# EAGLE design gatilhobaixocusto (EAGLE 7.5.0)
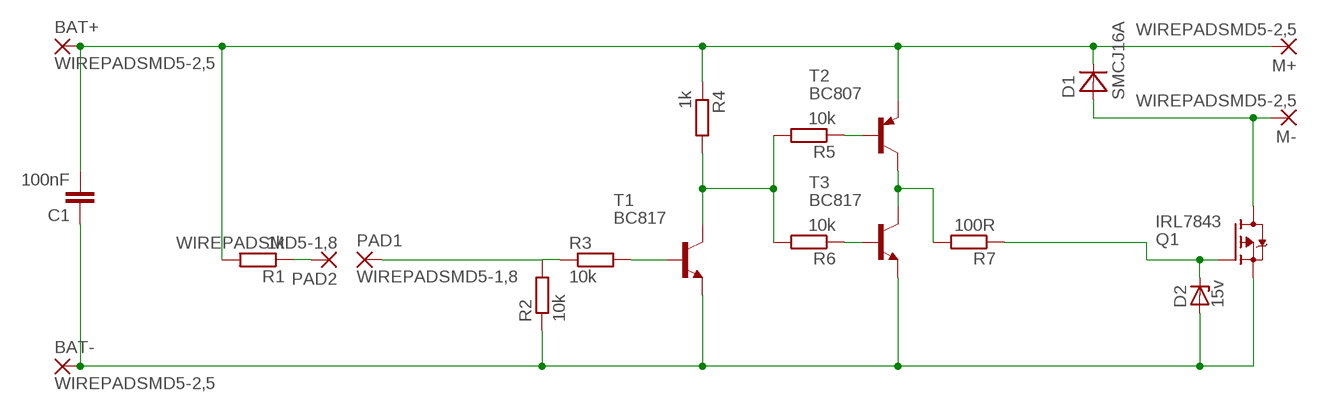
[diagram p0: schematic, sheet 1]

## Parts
BAT+  WIREPADSMD5-2,5  [5-2,5]
BAT-  WIREPADSMD5-2,5  [5-2,5]
C1  100nF  C-EUC0805K  [C0805K]
D1  SMCJ16A  MBRA340T3  [SMA]
D2  15v  ZENER-DIODESOD80C  [SOD80C]
M+  WIREPADSMD5-2,5  [5-2,5]
M-  WIREPADSMD5-2,5  [5-2,5]
PAD1  WIREPADSMD5-1,8  [5-1,8]
PAD2  WIREPADSMD5-1,8  [5-1,8]
Q1  IRL7843  FDD4141TO252  [TO252]
R1  1k  R-EU_R0805  [R0805]
R2  10k  R-EU_R0805  [R0805]
R3  10k  R-EU_R0805  [R0805]
R4  1k  R-EU_R0805  [R0805]
R5  10k  R-EU_R0805  [R0805]
R6  10k  R-EU_R0805  [R0805]
R7  100R  R-EU_R0805  [R0805]
T1  BC817  MMBT3904LT1-NPN-SOT23-BEC  [SOT23-BEC]
T2  BC807  MMBT3906LT1-PNP-SOT23-BEC  [SOT23-BEC]
T3  BC817  MMBT3904LT1-NPN-SOT23-BEC  [SOT23-BEC]

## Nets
N$1: BAT-.1(P) C1.1 D2.A Q1.2(S) R2.1 T1.E T3.E
N$2: D1.A M-.1(P) Q1.3(D)
N$4: PAD2.1(P) R1.1
N$5: BAT+.1(P) C1.2 D1.C M+.1(P) R1.2 R4.1 T2.E
N$7: PAD1.1(P) R2.2 R3.1
N$11: R4.2 R5.2 R6.2 T1.C
N$12: R3.2 T1.B
N$13: R7.2 T2.C T3.C
N$15: R5.1 T2.B
N$16: R6.1 T3.B
N$17: D2.C Q1.1(G) R7.1

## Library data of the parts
BAT+ BAT- M+ M- PAD1 PAD2 = wirepad:WIREPAD: Wire PAD connect wire on PCB
C1 = rcl:C-EU: CAPACITOR, European symbol
D1 = diode:MBRA340T3: Surface Mount Schottky Power Rectifier
D2 = diode:ZENER-DIODE: Z-Diode
Q1 = transistor-fet:FDD4141: P-Channel PowerTrench® MOSFET Source: FDD4141.pdf
R1-R7 = resistor:R-EU_: RESISTOR, European symbol
T1 T3 = transistor-neu-to92:*-NPN-: NPN Transistror
T2 = transistor:*-PNP-: PNP Transistror

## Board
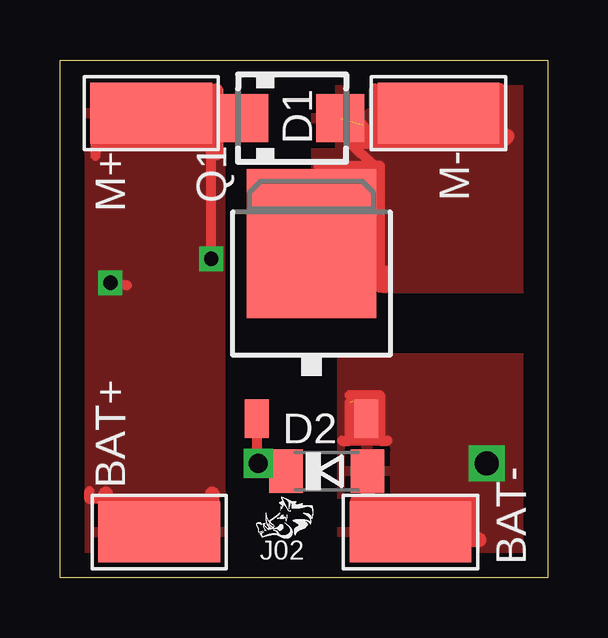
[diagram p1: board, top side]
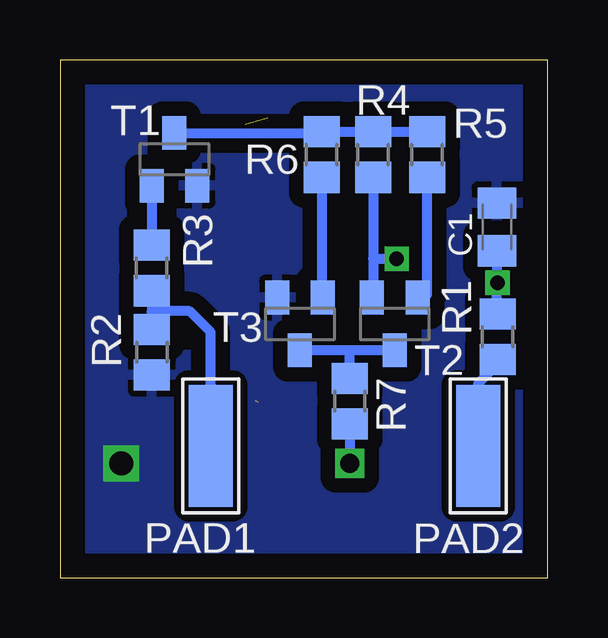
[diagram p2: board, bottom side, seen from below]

Size 20.33 x 21.59 mm. Coordinates in mm from the lower left corner, seen from the top.
Outline: 20.32,21.59 0,21.59 0,0 20.32,0
Outline: 20.33,21.59 20.33,0
Copper layers (1*16): Top 0.035mm / dielectric 1.5mm / Bottom 0.035mm
Design rules "default": minimum track width 10mil, minimum drill 24mil, track to track 8mil, track to pad 8mil, pad to pad 8mil, via to via 8mil, smd to smd 8mil, copper to edge 40mil, drill to drill 8mil, minimum pad ring 10mil, minimum via ring 8mil, stop-mask expansion 4mil, vias tented up to drill 0mil, thermal gap 10mil

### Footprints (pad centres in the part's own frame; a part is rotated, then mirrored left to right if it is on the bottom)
5-2,5 = smd 2.54 x 5.08: 1 0,0
C0805K = smd 1.3 x 1.6: 1 -1,0; 2 1,0
SMA = smd 2 x 2: A 2,0; C -2,0
SOD80C = smd 1.4 x 1.8: A 1.7,0; C -1.7,0
5-1,8 = smd 1.829 x 5.08: 1 0,0
TO252 = smd 1 x 1.6: 1 -2.28,-4.8; 2 2.28,-4.8 | smd 5.4 x 6.2: 3 0,2.5
R0805 = smd 1.3 x 1.5: 1 -0.95,0; 2 0.95,0
SOT23-BEC = smd 1 x 1.4: B -0.95,-1.1; C 0,1.1; E 0.95,-1.1

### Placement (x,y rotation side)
BAT+  4.13,1.91 90 top
BAT-  14.61,1.91 270 top
C1  2.12,14.63 270 bottom
D1  9.67,19.16 0 top
D2  11.11,4.45 0 top
M+  3.81,19.37 90 top
M-  15.77,19.37 270 top
PAD1  14.05,5.5 180 bottom
PAD2  2.9,5.5 0 bottom
Q1  10.48,11.43 0 top
R1  2.09,10.05 90 bottom
R2  16.5,9.4 90 bottom
R3  16.51,12.92 90 bottom
R4  7.29,17.65 90 bottom
R5  5.03,17.65 90 bottom
R6  9.43,17.65 90 bottom
R7  8.26,7.36 90 bottom
T1  15.56,17.45 0 bottom
T2  6.38,10.58 180 bottom
T3  10.33,10.58 180 bottom

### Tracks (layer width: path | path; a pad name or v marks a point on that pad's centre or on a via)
N$1  (via drill 1)  (1 unrouted)
  Top 0.406: 13.34,5.71 13.65,5.71 | 12.06,7.62 13.34,7.62 13.34,5.71 | 13.34,5.71 12.06,5.71 | 12.06,5.71 12.06,7.3 | 11.75,5.71 12.06,5.71 | 12.19,7.37 12.19,7.11
  Top 0.61: 12.38,3.17 12.7,3.17 | 12.7,3.17 17.14,3.17 17.14,1.59 | D2.A 12.81,3.29 12.7,3.17 | 17.14,1.59 17.46,1.59 | 16.83,1.59 17.14,1.59
  other vias: 17.78,4.76
  pour Top: 11.75,0.32 19.37,0.32 19.37,9.14 11.75,9.14
  pour Bottom (isolate 0.61): 19.37,21.27 19.37,0.32 0.64,0.32 0.64,21.27
N$2  (1 unrouted)
  Top 0.406: 10.78,17.18 13.12,17.18 | 12.87,12.69 12.87,12.78 13.6,12.8 13.58,12.08 13.33,12.08 13.33,17.18 13.12,17.18 | 13.1,20.4 13.1,18.4 12.91,18.59 | 13.12,17.18 12.1,18.1 13.3,18.1 | 12.91,18.41 12.91,18.59 | 12.91,18.59 12.6,18.9
  Top 0.61: 18.31,18.1 13.3,18.1 13.23,18.1 13.23,18.41 12.91,18.41 | 18.31,18.1 18.31,20.32 | 18.63,18.41 18.31,18.1
  pour Top: 10.66,21.27 10.64,12.08 19.37,12.08 19.37,21.27
N$4
  Bottom 0.406: PAD2.1 2.9,8.11 2.1,8.9 R1.1
N$5  (via drill 0.6)
  Top 0.406: 1.77,18.25 1.47,18.25 1.47,17.59 | 2.23,3.29 1.22,3.29 1.22,3.61 | 1.5,18 5.5,18 | 5.5,18 6.1,18 | 6.1,18 6.2,18 6.2,17.9 | v6.3,13.3 6.3,17.8 | 6.3,17.8 6.1,18 | D1.C 5.44,19.16 5,19.6 5,18.5 5.5,18 | 6.3,17.8 6.5,17.8 | v2.1,12.3 2.8,12.2
  Top 0.61: 6.35,3.17 4.45,3.17 | 4.45,3.17 1.91,3.17 | BAT+.1 4.13,2.86 4.45,3.17 | 1.91,3.17 1.91,3.49 | 1.91,3.17 1.91,2.86 | 6.35,3.17 6.35,3.49 | 6.35,3.17 6.35,2.86 | 6.5,20.3 6.5,17.8 6.5,17.7
  Bottom 0.406: R4.1 7.29,13.3 | 7.29,13.3 7.29,11.74 T2.E | 7.29,13.3 v6.3,13.3 | R1.2 2.12,11.63 2.12,12.18 v2.1,12.3 2.12,12.22 C1.2
  pour Top: 0.64,0.32 0.64,21.27 6.67,21.27 6.67,0.32
N$7
  Bottom 0.406: R3.1 16.51,11.1 | 16.51,11.1 R2.2 | 16.51,11.1 16.5,11.11 14.92,11.11 14.05,10.24 PAD1.1
N$11
  Bottom 0.406: 15.56,18.09 T1.C 9.38,18.55 R6.2 R4.2 R5.2
N$12
  Bottom 0.406: T1.B 16.51,13.97 R3.2
N$13
  Bottom 0.406: T2.C 8.3,9.48 | 8.3,9.48 T3.C | R7.2 8.26,9.44 8.3,9.48
N$15
  Bottom 0.406: R5.1 5.03,11.79 5.32,11.79 T2.B
N$16
  Bottom 0.406: R6.1 9.43,11.74 T3.B
N$17  (via drill 0.8)
  Top 0.406: Q1.1 8.2,4.82 v8.26,4.76 8.57,4.45 D2.C
  Bottom 0.406: R7.1 v8.26,4.76

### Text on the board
tPlace: J02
